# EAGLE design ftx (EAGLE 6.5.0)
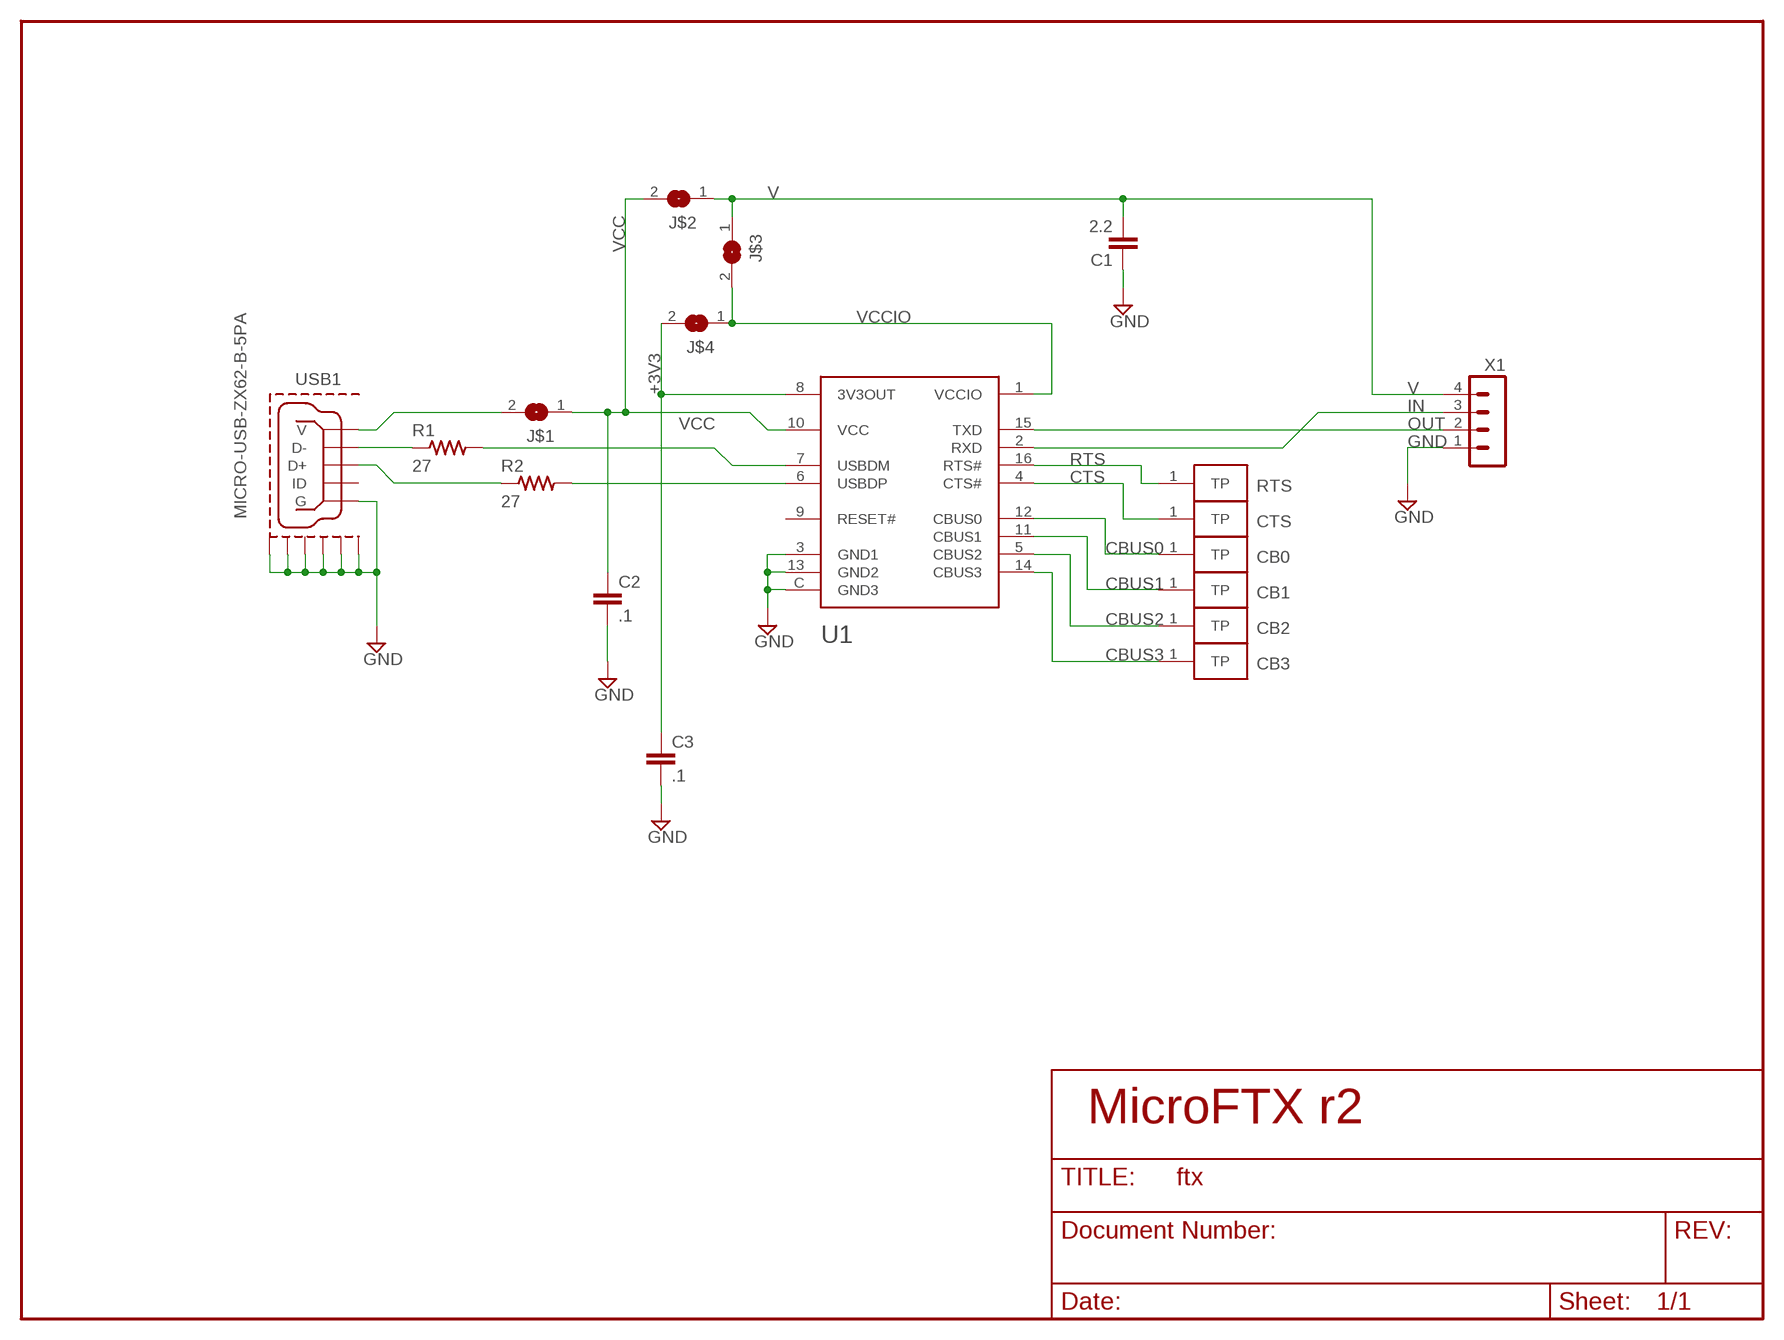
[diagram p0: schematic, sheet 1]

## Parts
C1  2.2  CAP0402  [SMD0402]
C2  .1  CAP0402  [SMD0402]
C3  .1  CAP0402  [SMD0402]
CB0  TESTPOINTHOLE  TESTPOINTBIG  [MA01-1]
CB1  TESTPOINTHOLE  TESTPOINTBIG  [MA01-1]
CB2  TESTPOINTHOLE  TESTPOINTBIG  [MA01-1]
CB3  TESTPOINTHOLE  TESTPOINTBIG  [MA01-1]
CTS  TESTPOINTHOLE  TESTPOINTBIG  [MA01-1]
J$1  SJJIM  [SJ_2_ROUND]
J$2  SJJIM  [SJ_2_ROUND]
J$3  SJJIM  [SJ_2_ROUND]
J$4  SJJIM  [SJ_2_ROUND]
R1  27  RES0402  [SMD0402]
R2  27  RES0402  [SMD0402]
RTS  TESTPOINTHOLE  TESTPOINTBIG  [MA01-1]
U1  FT230XQ  [QFN4X4-16]
USB1  MICRO-USB-ZX62-B-5PA  [ZX62-B-5PA]
X1  MA04-1  [MA04-1]

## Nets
+3V3: C3.1 J$4.2 U1.8(3V3OUT)
CBUS0: CB0.1(TP) U1.12(CBUS0)
CBUS1: CB1.1(TP) U1.11(CBUS1)
CBUS2: CB2.1(TP) U1.5(CBUS2)
CBUS3: CB3.1(TP) U1.14(CBUS3)
CTS: CTS.1(TP) U1.4(CTS#)
D+: R2.1 USB1.3(D+)
GND [power]: C1.1 C2.2 C3.2 U1.3(GND1) U1.13(GND2) U1.C(GND3) USB1.5(G) USB1.GND@1(GND1) USB1.GND@2(GND2) USB1.GND@3(GND3) USB1.GND@4(GND4) USB1.GND@5(GND5) USB1.GND@6(GND6) X1.1
IN: U1.2(RXD) X1.3
N$1: R1.1 USB1.2(D-)
OUT: U1.15(TXD) X1.2
RTS: RTS.1(TP) U1.16(RTS#)
USBDM: R1.2 U1.7(USBDM)
USBDP: R2.2 U1.6(USBDP)
V [power]: C1.2 J$2.1 J$3.1 X1.4
VBUS [power]: J$1.2 USB1.1(V)
VCC [power]: C2.1 J$1.1 J$2.2 U1.10(VCC)
VCCIO: J$3.2 J$4.1 U1.1(VCCIO)
Unconnected: U1.9(RESET#) USB1.4(ID)

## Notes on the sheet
- MicroFTX r2

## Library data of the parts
C1-C3 = serial:CAP
CB0 CB1-CB3 CTS RTS = serial:TESTPOINT
J$1-J$4 = serial:SJ: SMD solder JUMPER
R1 R2 = serial:RES
U1 = serial:FT230XQ
USB1 = serial:MICRO-USB: MICRO USB B, BOTTOM MOUNT
X1 = serial:MA04-1: PIN HEADER

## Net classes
1 power: width 0.305 mm

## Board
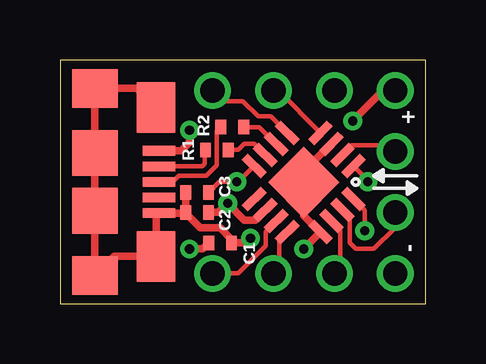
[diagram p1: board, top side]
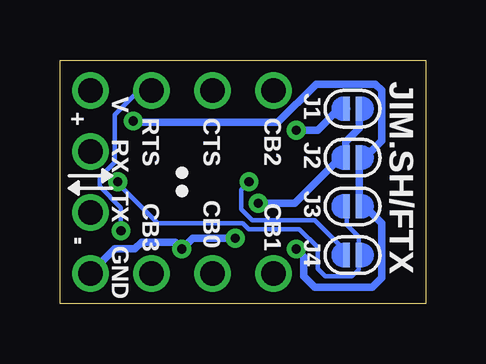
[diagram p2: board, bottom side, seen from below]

Size 15.24 x 10.16 mm. Coordinates in mm from the lower left corner, seen from the top.
Outline: 0,0 15.24,0 15.24,10.16 0,10.16 0,0
Copper layers (1*16): Top 0.0356mm / dielectric 1.5011mm / Bottom 0.0356mm
Design rules "ftdi *": minimum track width 6mil, minimum drill 15mil, track to track 6mil, track to pad 6mil, pad to pad 6mil, via to via 6mil, smd to smd 6mil, copper to edge 10mil, drill to drill 10mil, minimum pad ring 10mil, minimum via ring 8mil, stop-mask expansion 4mil, vias tented up to drill 15mil, thermal gap 10mil

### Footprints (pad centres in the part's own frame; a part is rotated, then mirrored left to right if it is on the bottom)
SMD0402 = smd 0.45 x 0.6: 1 -0.475,0; 2 0.475,0
MA01-1 = drill 1.016: 1 0,0
SJ_2_ROUND = smd 0.254 x 1.016: 1 -0.254,0; 2 0.254,0
QFN4X4-16 = smd 1.1 x 0.35: 1 -1.95,0.975; 2 -1.95,0.325; 3 -1.95,-0.325; 4 -1.95,-0.975; 9 1.95,-0.975; 10 1.95,-0.325; 11 1.95,0.325; 12 1.95,0.975 | smd 0.35 x 1.1: 5 -0.975,-1.95; 6 -0.325,-1.95; 7 0.325,-1.95; 8 0.975,-1.95; 13 0.975,1.95; 14 0.325,1.95; 15 -0.325,1.95; 16 -0.975,1.95 | smd 2.1 x 2.1: C 0,0
ZX62-B-5PA = smd 0.4 x 1.35: 1 -1.3,2.675; 2 -0.65,2.675; 3 0,2.675; 4 0.65,2.675; 5 1.3,2.675 | smd 2.1 x 1.6: GND@1 -3.1,2.55; GND@2 3.1,2.55 | smd 1.6 x 1.9: GND@3 3.9,0; GND@6 -3.9,0 | smd 1.9 x 1.9: GND@4 1.2,0; GND@5 -1.2,0
MA04-1 = drill 1.016: 1 -3.81,0; 2 -1.27,0; 3 1.27,0; 4 3.81,0

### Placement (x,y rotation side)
C1  6.67,2.54 180 top
C2  5.71,3.81 180 top
C3  5.71,4.64 180 top
CB0  8.89,1.27 0 bottom
CB1  6.35,1.27 0 bottom
CB2  6.35,8.89 0 bottom
CB3  11.43,1.27 0 bottom
CTS  8.89,8.89 0 bottom
J$1  3.05,8.13 180 bottom
J$2  3.05,6.1 180 bottom
J$3  3.05,4.06 180 bottom
J$4  3.05,2.03 180 bottom
R1  6.54,6.41 0 top
R2  7.18,7.37 0 top
RTS  11.43,8.89 0 bottom
U1  10.16,5.06 225 top
USB1  1.45,5.08 270 top
X1  13.97,5.08 90 top

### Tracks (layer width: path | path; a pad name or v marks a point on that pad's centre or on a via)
+3V3  (via drill 0.38)
  Top 0.178: U1.8 7.42,5.08 v7.37,5.08 6.63,5.08 C3.1
  Bottom 0.178: v7.37,5.08 7.68,4.76 7.68,3.94 7.24,3.49 4.64,3.49 3.3,2.16 J$4.2
CBUS0
  Top 0.178: CB0.1 9.14,1.52 9.14,2.6 9.47,2.93 U1.12
CBUS1
  Top 0.178: U1.11 8.57,3.01 8.57,2.41 7.43,1.27 CB1.1
CBUS2
  Top 0.178: U1.5 8.79,7.81 8.26,7.81 7.62,8.45 6.79,8.45 CB2.1
CBUS3
  Top 0.178: U1.14 11.68,3.07 11.68,1.52 CB3.1
CTS
  Top 0.178: CTS.1 9.09,8.89 U1.4
D+
  Top 0.178: USB1.3 4.7,5.08 4.95,5.33 6.1,5.33 6.54,5.78 6.54,7.21 R2.1
GND  (via drill 0.38)
  Top 0.305: C2.2 C3.2 | v10.16,2.29 10.85,2.98 U1.13 10.16,3.68 U1.C 10.16,5.52 U1.3 | USB1.GND@3 1.59,1.32 | 1.59,1.32 2.25,1.98 USB1.GND@2 4,3.65 USB1.5 5.21,3.78 | 1.59,1.32 1.45,1.47 USB1.GND@4 USB1.GND@5 USB1.GND@6 3.2,8.98 USB1.GND@1 | 5.21,3.78 5.27,3.78 | C2.2 5.24,3.78 5.84,3.17 6.67,3.17 7.14,2.7 C1.1 | C1.1 7.75,2.54 v7.94,2.73 | C1.1 7.14,2.51 | C2.2 5.21,3.78
  Bottom 0.305: X1.1 12.95,2.29 12.13,2.29 11.84,2.57 10.45,2.57 v10.16,2.29 9.72,2.73 v7.94,2.73
IN
  Top 0.178: U1.2 12.16,6.6 13.72,6.6 X1.3
N$1
  Top 0.178: USB1.2 5.92,5.73 6.03,5.84 6.03,6.38 R1.1
OUT
  Top 0.178: U1.15 12.06,3.61 12.06,2.54 12.32,2.29 13.08,2.29 13.97,3.17 X1.2
RTS  (via drill 0.38)
  Top 0.178: U1.16 12.7,3.9 v12.7,3.05
  Bottom 0.178: RTS.1 11.94,8.89 12.95,7.87 12.95,5.91 13.59,5.27 13.59,4.89 12.7,4 v12.7,3.05
USBDM
  Top 0.178: R1.2 7.43,6.41 7.68,6.67 8.09,6.67 U1.7
USBDP
  Top 0.178: R2.2 8.31,7.37 U1.6
V  (via drill 0.38)
  Top 0.305: v12.19,7.62 13.46,8.89 X1.4 | C1.2 5.94,2.29 v5.4,2.29
  Bottom 0.178: J$2.1 2.71,6.01 2.71,5.93 | 2.29,3.81 2.54,3.81 J$3.1
  Bottom 0.305: v12.19,7.62 12.13,7.56 6.16,7.56 4.57,9.14 2.1,9.14 1.84,8.89 1.84,6.79 2.71,5.93 2.77,5.87 2.77,4.34 2.51,4.09 2.51,3.86 2.33,3.86 2.29,3.81 1.84,3.37 1.84,1.08 2.22,0.7 4.64,0.7 5.08,1.14 5.08,1.97 v5.4,2.29
VBUS  (via drill 0.38)
  Top 0.305: USB1.1 5.05,6.38 5.4,6.73 v5.4,7.24
  Bottom 0.305: J$1.2 3.62,8.13 4.51,7.24 v5.4,7.24
VCC  (via drill 0.38)
  Top 0.305: C2.1 6.6,3.81 v6.99,4.19 7.68,3.49 8.13,3.49 8.26,3.62 U1.10
  Bottom 0.178: 2.74,8.13 J$1.1 2.56,8.13 | 3.33,6.33 3.3,6.3 J$2.2
  Bottom 0.305: v6.99,4.19 5.46,4.19 3.33,6.33 3.33,6.76 2.77,7.32 2.77,7.75 2.56,7.95 2.56,8.13
VCCIO  (via drill 0.38)
  Top 0.178: v12.83,5.08 12.83,5.15 U1.1
  Bottom 0.178: v12.83,5.08 12.83,5.02 11.18,3.37 7.62,3.37 7.37,3.11 5.27,3.11 4.51,2.35 4.51,1.46 4.19,1.14 3.07,1.14 2.79,1.42 J$4.1 2.79,2.79 3.3,3.3 J$3.2

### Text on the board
tNames: + | -
bNames: JIM.SH/FTX | J1 | V | + | J2 | RX | J3 | TX | J4 | - | GND
tSilk: R2 | + | R1 | C3 | C2 | C1 | -
bSilk: JIM.SH/FTX | J1 | V | CB2 | CTS | RTS | + | J2 | RX | J3 | TX | CB1 | CB0 | CB3 | J4 | - | GND
_tnames: R2 | + | R1 | C3 | C2 | C1 | -
_bnames: JIM.SH/FTX | J1 | V | CB2 | CTS | RTS | + | J2 | RX | J3 | TX | CB1 | CB0 | CB3 | J4 | - | GND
